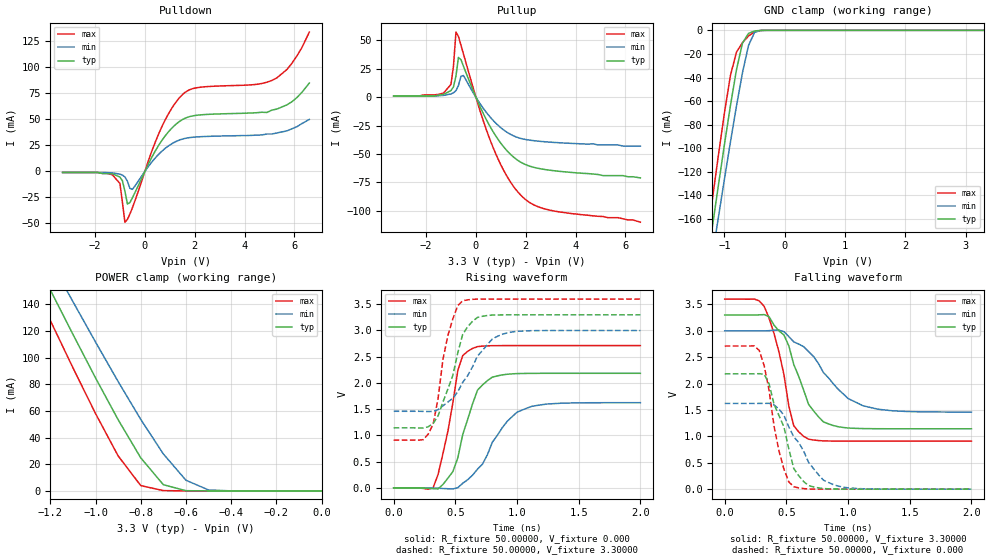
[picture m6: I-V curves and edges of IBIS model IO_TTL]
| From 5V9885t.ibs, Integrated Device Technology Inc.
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|   Model IO_TTL
[Model]   IO_TTL
Model_type   3-state
Polarity   Non-Inverting
Enable   Active-High
Vmeas =  1.65000V
C_comp   5.10000pF   5.10000pF   5.10000pF
[Temperature Range]   25.00000   100.00000   -40.00000
[Voltage Range]   3.30000V   3.00000V   3.60000V
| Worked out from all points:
|   slope of the pulldown table from 0 to 0.495 V, typ, clamps not added: 21.7 ohm
|   slope of the pullup table from 0 to 0.495 V, typ, clamps not added: 21.7 ohm
|   GND clamp passes 1 mA (typ) near -0.52 V on its own axis
|   POWER clamp passes 1 mA (typ) near -0.62 V on its own axis
|   rising waveform, R_fixture 50.00000, V_fixture 0.000: 20-80 % time 163ps typ, 266ps min, 127ps max; typ from 0 V to 2.18 V
|   rising waveform, R_fixture 50.00000, V_fixture 3.30000: 20-80 % time 163ps typ, 247ps min, 120ps max; typ from 1.14 V to 3.3 V
|   falling waveform, R_fixture 50.00000, V_fixture 3.30000: 20-80 % time 200ps typ, 334ps min, 149ps max; typ from 3.3 V to 1.14 V
|   falling waveform, R_fixture 50.00000, V_fixture 0.000: 20-80 % time 169ps typ, 244ps min, 127ps max; typ from 2.19 V to 0 V
[Pulldown]
| voltage   I(typ)   I(min)   I(max)
-3.3V     -1mA       -1mA       -1mA
-1.3V     -2.3mA     -1.4mA     -3.3mA
-1V       -5.4mA     -2.6mA     -11.6mA
-800mV    -19.08mA   -5.3mA     -48.82mA
-700mV    -31.3mA    -9.44mA    -46.17mA
-600mV    -29.94mA   -16.29mA   -40.99mA
600mV     26.79mA    17.54mA    38.63mA
1.5V      49.75mA    31.08mA    73.68mA
2.1V      54.05mA    33.2mA     80.54mA
5.1V      59mA       36mA       87.5mA
5.9V      67mA       41mA       104mA
6.6V      85mA       50mA       134mA
[Pullup]
| voltage   I(typ)   I(min)   I(max)
-3.3V     1mA        1mA        1mA
-1.3V     2.5mA      1.6mA      3.6mA
-1V       5.9mA      2.9mA      11.3mA
-900mV    9.1mA      3.9mA      27.28mA
-800mV    18.66mA    5.8mA      57.34mA
-700mV    35.02mA    10.29mA    53.48mA
-600mV    33.03mA    18.46mA    45.88mA
600mV     -26.97mA   -18.17mA   -39.29mA
1.2V      -45.91mA   -30.14mA   -67.81mA
1.8V      -57.19mA   -36.25mA   -86.19mA
2.9V      -64.05mA   -39.43mA   -99.04mA
6.6V      -71mA      -43mA      -110mA
[GND_clamp]
| voltage   I(typ)   I(min)   I(max)
-3.3V     -941mA     -907.6mA   -976.3mA
-1.3V     -202.4mA   -224.6mA   -181.6mA
-1.2V     -166.7mA   -191.4mA   -143.4mA
-1.1V     -131.5mA   -158.6mA   -106mA
-1V       -96.95mA   -126.3mA   -70.13mA
-900mV    -63.73mA   -94.63mA   -38.18mA
-800mV    -33.34mA   -64.12mA   -18.46mA
-700mV    -10.74mA   -35.84mA   -10.48mA
-600mV    -2.575mA   -12.79mA   -4.779mA
-500mV    -539.2uA   -1.691mA   -1.235mA
-400mV    -63.39uA   -109.7uA   -138.9uA
3.3V      1.113nA    1.554uA    594.4pA
[POWER_clamp]
| voltage   I(typ)   I(min)   I(max)
-3.3V     883.3mA    846.6mA    910.2mA
-1.3V     184.6mA    203.9mA    164mA
-1.2V     150.8mA    172.8mA    127.9mA
-1.1V     117.5mA    142mA      92.41mA
-1V       84.79mA    111.7mA    58.08mA
-900mV    53.43mA    82.04mA    26.28mA
-800mV    24.83mA    53.65mA    4.001mA
-700mV    4.655mA    27.71mA    235uA
-600mV    173.3uA    7.999mA    25.91uA
-500mV    5.672uA    712.7uA    2.386uA
-400mV    254.7nA    34.2uA     117.2nA
0V        1.113nA    3.548nA    890.2pA
[Ramp]
| variable   typ   min   max
dV/dt_r   1.31040/0.16413n   0.97440/0.25535n   1.62720/0.11213n
dV/dt_f   1.29360/0.20881n   0.92400/0.33333n   1.61394/0.14020n
R_load = 50.00000
[Rising Waveform]
R_fixture = 50.00000
V_fixture = 0.000
V_fixture_min = 0.000
V_fixture_max = 0.000
| time   V(typ)   V(min)   V(max)
0s        0V         0V         0V
320ps     -15.86mV   -1.699mV   3.863mV
440ps     185.5mV    -16.55mV   1.083V
520ps     572.3mV    3.505mV    2.236V
560ps     1.016V     87.9mV     2.522V
640ps     1.605V     242.1mV    2.659V
680ps     1.863V     358.2mV    2.692V
800ps     2.111V     870.4mV    2.711V
1ns       2.179V     1.442V     2.712V
2ns       2.184V     1.624V     2.712V
[Rising Waveform]
R_fixture = 50.00000
V_fixture = 3.30000
V_fixture_min = 3.00000
V_fixture_max = 3.60000
| time   V(typ)   V(min)   V(max)
0s        1.144V     1.46V      910mV
240ps     1.142V     1.458V     919.3mV
320ps     1.227V     1.459V     1.212V
400ps     1.641V     1.565V     2.454V
440ps     1.886V     1.637V     2.907V
520ps     2.576V     1.832V     3.474V
560ps     2.928V     2.013V     3.567V
680ps     3.25V      2.514V     3.599V
920ps     3.299V     2.955V     3.599V
2ns       3.299V     2.999V     3.599V
[Falling Waveform]
R_fixture = 50.00000
V_fixture = 3.30000
V_fixture_min = 3.00000
V_fixture_max = 3.60000
R_dut = 0.000
| time   V(typ)   V(min)   V(max)
0s        3.3V       3V         3.6V
320ps     3.307V     2.999V     3.465V
440ps     2.999V     3.013V     2.598V
520ps     2.714V     2.891V     1.573V
560ps     2.361V     2.791V     1.202V
640ps     1.877V     2.7V       1V
680ps     1.607V     2.608V     947.3mV
800ps     1.276V     2.211V     914.6mV
1.12ns    1.148V     1.581V     910.2mV
2ns       1.144V     1.46V      910.1mV
[Falling Waveform]
R_fixture = 50.00000
V_fixture = 0.000
V_fixture_min = 0.000
V_fixture_max = 0.000
R_dut = 0.000
| time   V(typ)   V(min)   V(max)
0s        2.185V     1.624V     2.712V
280ps     2.188V     1.625V     2.628V
360ps     1.994V     1.626V     1.868V
440ps     1.395V     1.518V     724.2mV
480ps     1.181V     1.399V     381.3mV
520ps     760.1mV    1.179V     136.6mV
560ps     390.2mV    991.1mV    47.23mV
760ps     23.99mV    275mV      990.1uV
920ps     2.33mV     58.18mV    223.4uV
2ns       89.17uV    114.2uV    69.17uV
